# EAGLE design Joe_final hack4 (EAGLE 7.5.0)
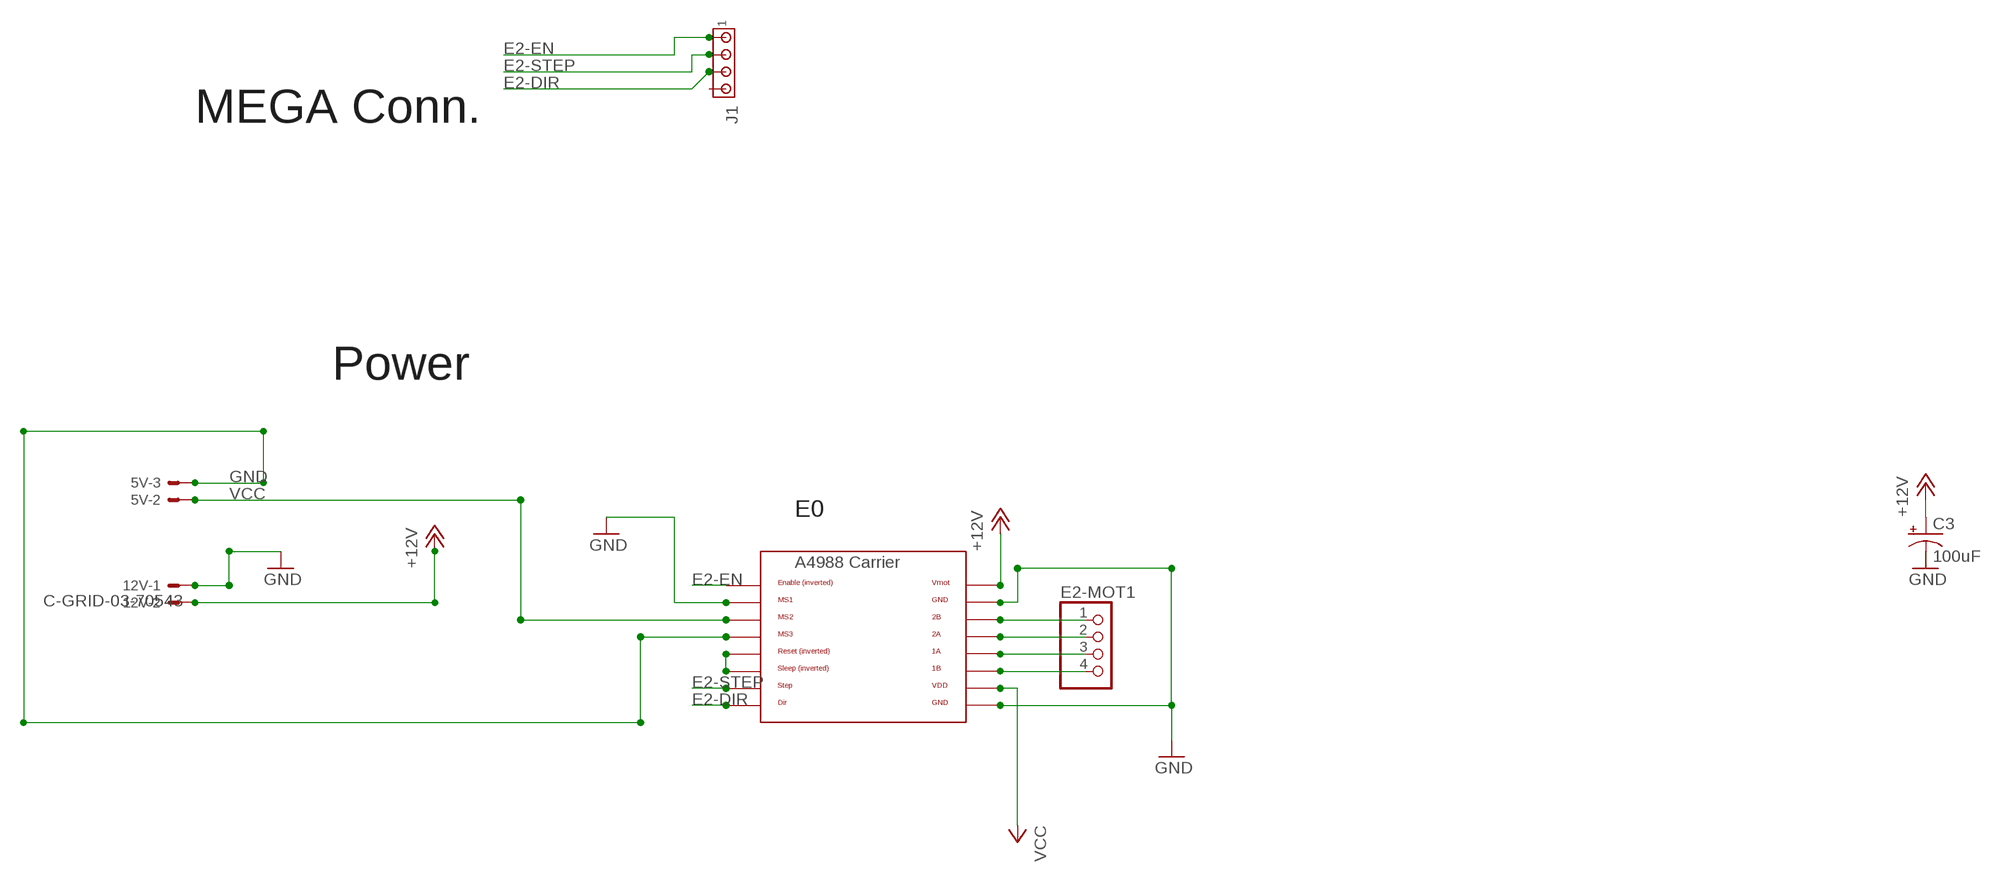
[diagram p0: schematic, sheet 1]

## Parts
5V  C-GRID-03-70543  [70543-03]
12V  C-GRID-03-70543  [70543-03]
C3  100uF  CPOL-US153CLV-0605  [153CLV-0605]
E2-MOT1  PINHD-1X4  [1X04]
J1  MTA04-156  [1X4MTA]
U$4  A4988BREAKOUT  [A4988BREAKOUT]

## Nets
+12V: 12V.2 C3.+ U$4.VMOT
E2-DIR: J1.3 U$4.DIR
E2-EN: J1.1 U$4.EN
E2-STEP: J1.2 U$4.STEP
GND: 5V.3 12V.1 C3.- U$4.GND U$4.GND@0(GND) U$4.MS1 U$4.MS3
N$4: E2-MOT1.1 U$4.2B
N$8: U$4.RST U$4.SLP(SLEEP)
N$10: E2-MOT1.2 U$4.2A
N$11: E2-MOT1.3 U$4.1A
N$12: E2-MOT1.4 U$4.1B
VCC: 5V.2 U$4.MS2 U$4.VDD
Unconnected: 5V.1 12V.3 J1.4

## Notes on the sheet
- MEGA Conn.
- Power
- E0

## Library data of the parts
5V 12V = con-molex:C-GRID-03: CONNECTOR wire to board 2.54 mm (0.100") pitch header; OC_FARNELL: unknown; OC_NEWARK: unknown
C3 = adafruit:CPOL-US: POLARIZED CAPACITOR, American symbol
E2-MOT1 = RepRapjr:PINHD-1X4: PIN HEADER
J1 = con-amp:MTA04-156: AMP connector
U$4 = RepRapjr:A4988BREAKOUT

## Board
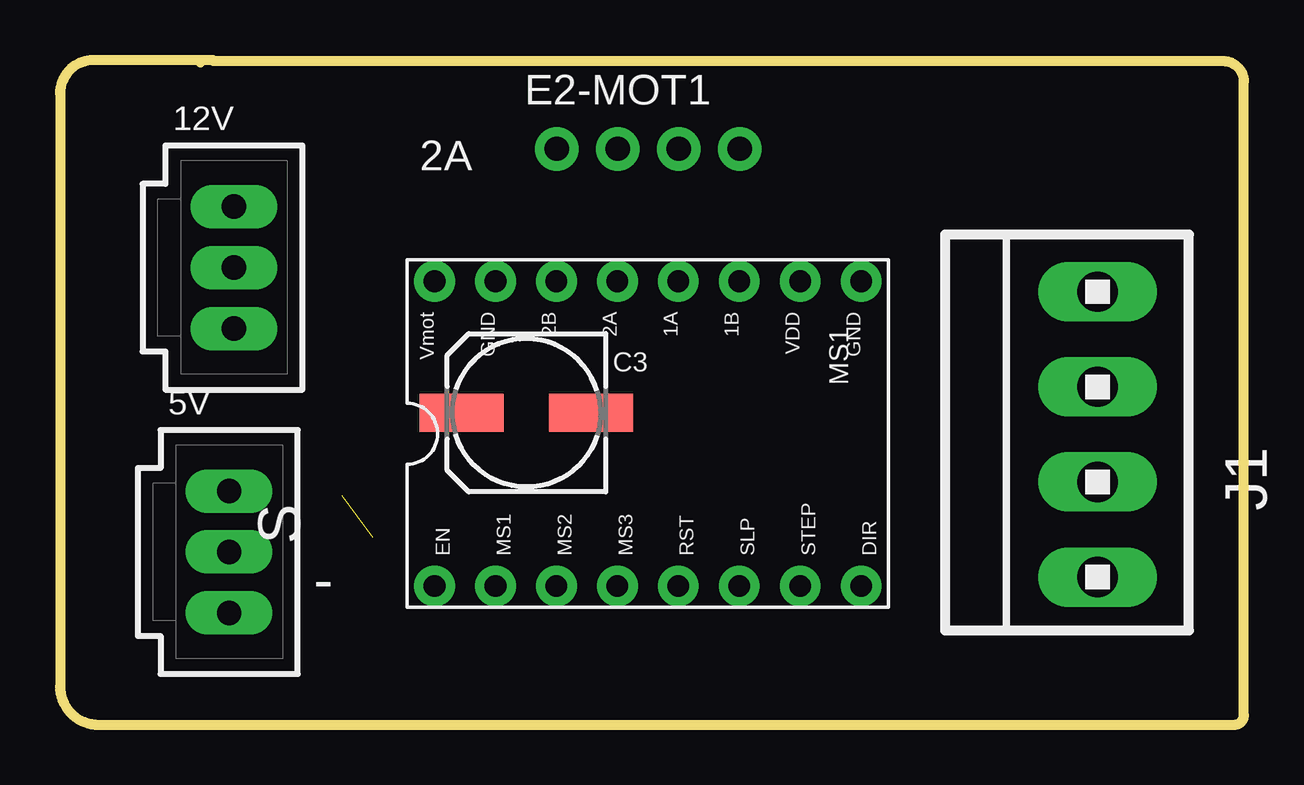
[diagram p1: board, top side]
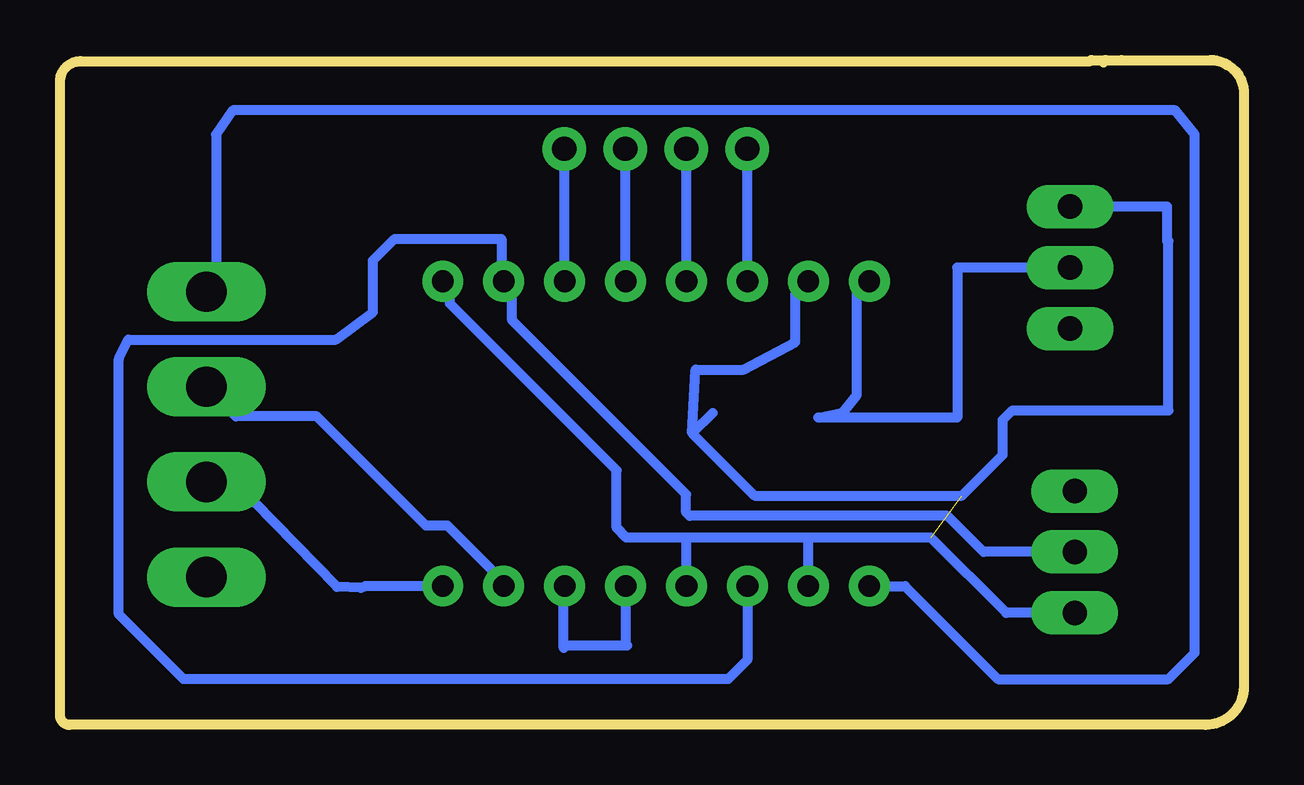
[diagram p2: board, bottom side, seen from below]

Size 49.35 x 27.7 mm. Coordinates in mm from the lower left corner, seen from the top.
Outline: 5.85,27.6 arc90 5.75,27.7
Outline: 5.75,27.7 5.1,27.7 1.4,27.7 arc90 0,26.3 0,1.6 arc90 1.6,0 48.95,0 arc90 49.35,0.4 49.35,26.8 arc90 48.5,27.65 6.4,27.65 arc90 6.35,27.7 5.75,27.7
Copper layers (1*16): Top 0.035mm / dielectric 1.6mm / Bottom 0.035mm
Design rules "PCB-CART *": minimum track width 0.1mm, minimum drill 0.1mm, track to track 16mil, track to pad 16mil, pad to pad 16mil, via to via 16mil, smd to smd 16mil, copper to edge 0.1mm, drill to drill 0.1mm, minimum pad ring 0.4mm, minimum via ring 0.3mm, stop-mask expansion 3mil, vias tented up to drill 0.5mm, thermal gap 12mil

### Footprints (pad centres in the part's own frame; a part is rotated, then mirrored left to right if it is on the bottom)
70543-03 = drill 1.016 long: 1 -2.54,0; 2 0,0; 3 2.54,0
153CLV-0605 = smd 3.5 x 1.6: + 2.7,0; - -2.7,0
1X04 = drill 1.016: 1 -2.54,0; 2 0,0; 3 2.54,0; 4 5.08,0
1X4MTA = drill 1.676 long: 1 5.944,0; 2 1.981,0; 3 -1.981,0; 4 -5.944,0
A4988BREAKOUT = drill 0.9: 1A 8.89,1.27; 1B 11.43,1.27; 2A 6.35,1.27; 2B 3.81,1.27; DIR 16.51,-11.43; EN -1.27,-11.43; GND 16.51,1.27; GND@0 1.27,1.27; MS1 1.27,-11.43; MS2 3.81,-11.43; MS3 6.35,-11.43; RST 8.89,-11.43; SLP 11.43,-11.43; STEP 13.97,-11.43; VDD 13.97,1.27; VMOT -1.27,1.27

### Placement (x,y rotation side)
5V  7.05,7.2 270 top
12V  7.25,19.05 270 top
C3  19.44,13 180 top
E2-MOT1  23.25,24 0 top
J1  43.25,12.1 90 top
U$4  16.88,17.21 0 top

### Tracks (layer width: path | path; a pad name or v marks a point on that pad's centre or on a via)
+12V
  Bottom 0.406: 12V.2 11.95,19.05 11.95,12.8 17.74,12.8 C3.+ 16.15,13.74 16.15,18.48 U$4.VMOT
E2-DIR
  Bottom 0.406: U$4.DIR 36.62,5.78 36.8,5.7 37.8,5.75 41.25,9.3 42.43,9.3 J1.3
E2-EN
  Bottom 0.406: U$4.EN 14.13,5.78 10.25,1.9 3.15,1.9 2.05,3 2.05,24.6 2.85,25.6 42.15,25.6 42.85,24.6 42.85,18.44 J1.1
E2-STEP
  Bottom 0.406: U$4.STEP 30.86,5.95 33.2,8.3 34.1,8.3 38.65,12.85 42.02,12.85 J1.2
GND  (1 unrouted)
  Bottom 0.406: C3.- 23,12.15 | 23,12.15 20.4,9.55 11.75,9.55 10.05,11.25 10.05,12.7 9.65,13.1 3.15,13.1 3.15,20.15 3.2,20.15 3.2,21.59 12V.1 | 23,12.15 22.85,14.8 20.85,14.8 18.7,15.95 18.7,17.93 U$4.GND@0 | 5V.3 9.91,4.66 13.05,7.8 18.05,7.8 | 18.05,7.8 23.1,7.8 | 23.1,7.8 25.75,7.8 26.15,8.2 26.15,10.6 33.1,17.55 33.1,18.18 U$4.GND | U$4.MS1 18.16,7.7 18.05,7.8 | U$4.MS3 23.23,7.66 23.1,7.8
N$4
  Bottom 0.406: U$4.2B 20.7,23.98 E2-MOT1.1
N$8
  Bottom 0.406: U$4.RST 25.77,3.38 25.7,3.3 28.25,3.3 28.35,3.2 28.35,5.74 U$4.SLP
N$10
  Bottom 0.406: U$4.2A 23.23,23.98 E2-MOT1.2
N$11
  Bottom 0.406: U$4.1A 25.77,23.98 E2-MOT1.3
N$12
  Bottom 0.406: U$4.1B 28.31,23.98 E2-MOT1.4
VCC
  Bottom 0.406: 5V.2 10.85,7.2 12.35,8.7 23.1,8.7 23.25,8.85 23.25,9.6 30.5,16.85 30.5,18.12 U$4.VDD 30.95,18.57 30.95,20.25 35.4,20.25 36.3,19.35 36.3,17.2 37.85,16.05 46.5,16.05 46.9,15.25 46.9,4.6 44.2,1.9 21.5,1.9 20.7,2.7 U$4.MS2

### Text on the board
tNames: 2A | MS1 | S | -
Holes: /x3 stepper expander
Document: RAMPS 1.4.2.1 (RepRap Arduino MEGA Pololu Shield) | reprap.org/wiki/RAMPS1.4 | Reversing input power, and inserting stepper drivers incorrectly will destroy electronics.
_tsilk: + | I2C | END STOPS | 21 | 1 | 20 | 1 | - | + | 1 | + | 1 | 1 | 1 | 1 | 1 | 1 | 1 | -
